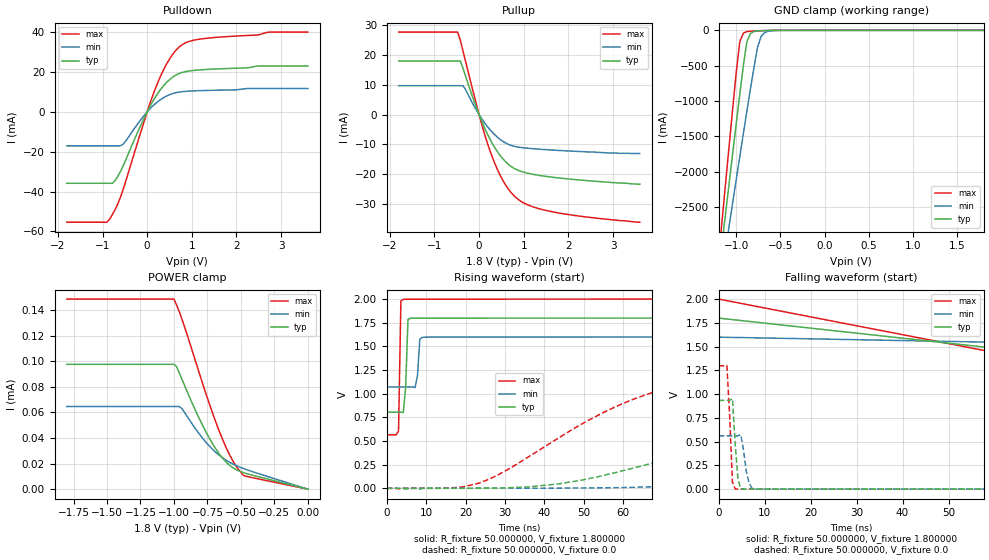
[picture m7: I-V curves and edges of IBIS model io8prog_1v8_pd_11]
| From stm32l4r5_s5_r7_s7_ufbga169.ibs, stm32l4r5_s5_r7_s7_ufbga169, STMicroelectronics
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|   Model io8prog_1v8_pd_11
[Model]  io8prog_1v8_pd_11
Model_type I/O
Polarity   Non-Inverting
Enable   Active-Low
Vinl =   0.540000V
Vinh =   1.260000V
Vmeas =  0.900000V
Cref =   100.000000nF
Rref =   1.000000k
Vref =   1.800000V
C_comp   2.197300pF   2.162700pF   2.264100pF
[Temperature Range]   25.000000   0.125000k   -40.000000
[Pullup Reference]   1.800000V   1.600000V   2.000000V
[Pulldown Reference]   0.0V   0.0V   0.0V
[POWER Clamp Reference]   1.800000V   1.600000V   2.000000V
[GND Clamp Reference]   0.0V   0.0V   0.0V
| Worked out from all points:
|   slope of the pulldown table from 0 to 0.27 V, typ, clamps not added: 26.2 ohm
|   slope of the pullup table from 0 to 0.27 V, typ, clamps not added: 30.1 ohm
|   GND clamp passes 1 mA (typ) near -0.58 V on its own axis
|   rising waveform, R_fixture 50.000000, V_fixture 1.800000: 20-80 % time 583ps typ, 535ps min, 376ps max; typ from 0.804 V to 1.8 V
|   rising waveform, R_fixture 50.000000, V_fixture 0.0: 20-80 % time 64.8ns typ, 104ns min, 36.2ns max; typ from 0 V to 0.934 V
|   falling waveform, R_fixture 50.000000, V_fixture 1.800000: 20-80 % time 115ns typ, 164ns min, 91.9ns max; typ from 1.8 V to 0.804 V
|   falling waveform, R_fixture 50.000000, V_fixture 0.0: 20-80 % time 811ps typ, 1.12ns min, 745ps max; typ from 0.934 V to 0 V
[Pulldown]
|Voltage   I(typ)   I(min)   I(max)
-1.8V     -35.82mA   -17.03mA   -55.35mA
-900mV    -35.82mA   -17.03mA   -55.35mA
-840mV    -35.82mA   -17.03mA   -53.76mA
-720mV    -34.49mA   -17.03mA   -49.08mA
-540mV    -27.18mA   -16.22mA   -39.07mA
-60mV     -2.756mA   -1.584mA   -4.227mA
240mV     9.353mA    5.171mA    14.85mA
480mV     15.75mA    8.427mA    25.77mA
720mV     19.29mA    9.947mA    32.62mA
960mV     20.57mA    10.43mA    35.5mA
1.32V     21.27mA    10.74mA    36.91mA
3.6V      23.04mA    11.73mA    40.04mA
[Pullup]
|Voltage   I(typ)   I(min)   I(max)
-1.8V     18.05mA    9.738mA    27.78mA
-480mV    18.05mA    9.738mA    27.78mA
-420mV    18.05mA    9.738mA    25.03mA
-360mV    15.57mA    9.738mA    21.38mA
60mV      -2.268mA   -1.401mA   -3.341mA
240mV     -8.143mA   -5.004mA   -12mA
360mV     -11.31mA   -6.914mA   -16.72mA
540mV     -15mA      -9.056mA   -22.31mA
840mV     -18.52mA   -10.83mA   -28.11mA
1.14V     -19.87mA   -11.38mA   -30.67mA
1.68V     -21.13mA   -11.96mA   -32.81mA
3.6V      -23.4mA    -13.1mA    -36.2mA
[GND_clamp]
|Voltage   I(typ)   I(min)   I(max)
-1.8V     -9.861A    -8.8A      -9.626A
-1.16V    -3.004A    -3.417A    -2.68A
-1.12V    -2.579A    -3.088A    -2.15A
-1.08V    -2.155A    -2.76A     -1.623A
-1V       -1.315A    -2.108A    -586.3mA
-960mV    -900.6mA   -1.784A    -158.3mA
-920mV    -496.8mA   -1.462A    -39.4mA
-880mV    -160.5mA   -1.144A    -17.83mA
-840mV    -45.94mA   -830.4mA   -12.53mA
-760mV    -8.275mA   -243mA     -7.558mA
-680mV    -3.402mA   -33.06mA   -3.844mA
1.8V      47.61uA    51.9uA     39.21uA
[POWER_clamp]
|Voltage   I(typ)   I(min)   I(max)
-1.8V     97.61uA    64.61uA    148.6uA
-1V       97.61uA    64.61uA    148.6uA
-980mV    95.77uA    64.61uA    143.9uA
-960mV    90.85uA    64.61uA    138.6uA
-940mV    85.82uA    62.87uA    132.7uA
-820mV    57.18uA    44.44uA    93.74uA
-720mV    36.98uA    32uA       61.96uA
-620mV    22.23uA    23.29uA    34.8uA
-560mV    16.76uA    19.67uA    22.06uA
-520mV    14.49uA    17.74uA    15.63uA
-480mV    12.91uA    16.08uA    10.62uA
0V        0A         0A         0A
[Ramp]
| variable   typ   min   max
dV/dt_r  0.56025/65.12955n   0.33658/0.11608u   0.77838/36.16086n
dV/dt_f  0.59723/66.14768n   0.31668/0.11599u   0.86050/35.16151n
R_load = 50.000000
[Rising Waveform]
R_fixture= 50.000000
V_fixture= 1.800000
V_fixture_min= 1.600000
V_fixture_max= 2.000000
|time   V(typ)   V(min)   V(max)
0s        804mV      1.071V     565.4mV
3.003ns   804.1mV    1.071V     605mV
3.604ns   804mV      1.071V     1.98V
4.204ns   800.5mV    1.071V     1.996V
4.805ns   1.063V     1.071V     1.997V
5.405ns   1.786V     1.071V     1.998V
6.006ns   1.796V     1.071V     1.998V
7.207ns   1.798V     1.065V     1.998V
9.61ns    1.798V     1.597V     1.998V
299.1ns   1.799V     1.599V     2V
[Rising Waveform]
R_fixture= 50.000000
V_fixture= 0.0
V_fixture_min= 0.0
V_fixture_max= 0.0
|time   V(typ)   V(min)   V(max)
0s        169uV      298.2uV    106.4uV
23.42ns   998.7uV    671.7uV    55.24mV
43.24ns   45.28mV    1.71mV     522.8mV
62.46ns   212.8mV    11.12mV    939.5mV
78.08ns   378.7mV    32.85mV    1.133V
94.89ns   544mV      75.69mV    1.225V
124.3ns   744.6mV    183.4mV    1.278V
156.8ns   853.9mV    303.1mV    1.292V
225.2ns   923.7mV    481.8mV    1.297V
299.1ns   933.9mV    561.3mV    1.297V
[Falling Waveform]
R_fixture= 50.000000
V_fixture= 1.800000
V_fixture_min= 1.600000
V_fixture_max= 2.000000
|time   V(typ)   V(min)   V(max)
0s        1.799V     1.599V     2V
150.2ns   1.007V     1.464V     593.9mV
300.3ns   817.1mV    1.136V     565.9mV
450.5ns   805.1mV    1.083V     565.4mV
750.8ns   804mV      1.072V     565.4mV
14.86us   804mV      1.071V     565.4mV
[Falling Waveform]
R_fixture= 50.000000
V_fixture= 0.0
V_fixture_min= 0.0
V_fixture_max= 0.0
|time   V(typ)   V(min)   V(max)
0s        933.9mV    561.3mV    1.297V
1.802ns   934.1mV    561.3mV    1.3V
2.402ns   934mV      561.3mV    771.5mV
3.003ns   952.3mV    561.4mV    75.96mV
3.604ns   478mV      561.5mV    3.458mV
4.204ns   106.3mV    561.2mV    1.049mV
4.805ns   5.486mV    574.3mV    708.6uV
6.607ns   692.9uV    69.79mV    625uV
7.808ns   615.4uV    2.085mV    615uV
299.1ns   169uV      298.2uV    106.4uV
